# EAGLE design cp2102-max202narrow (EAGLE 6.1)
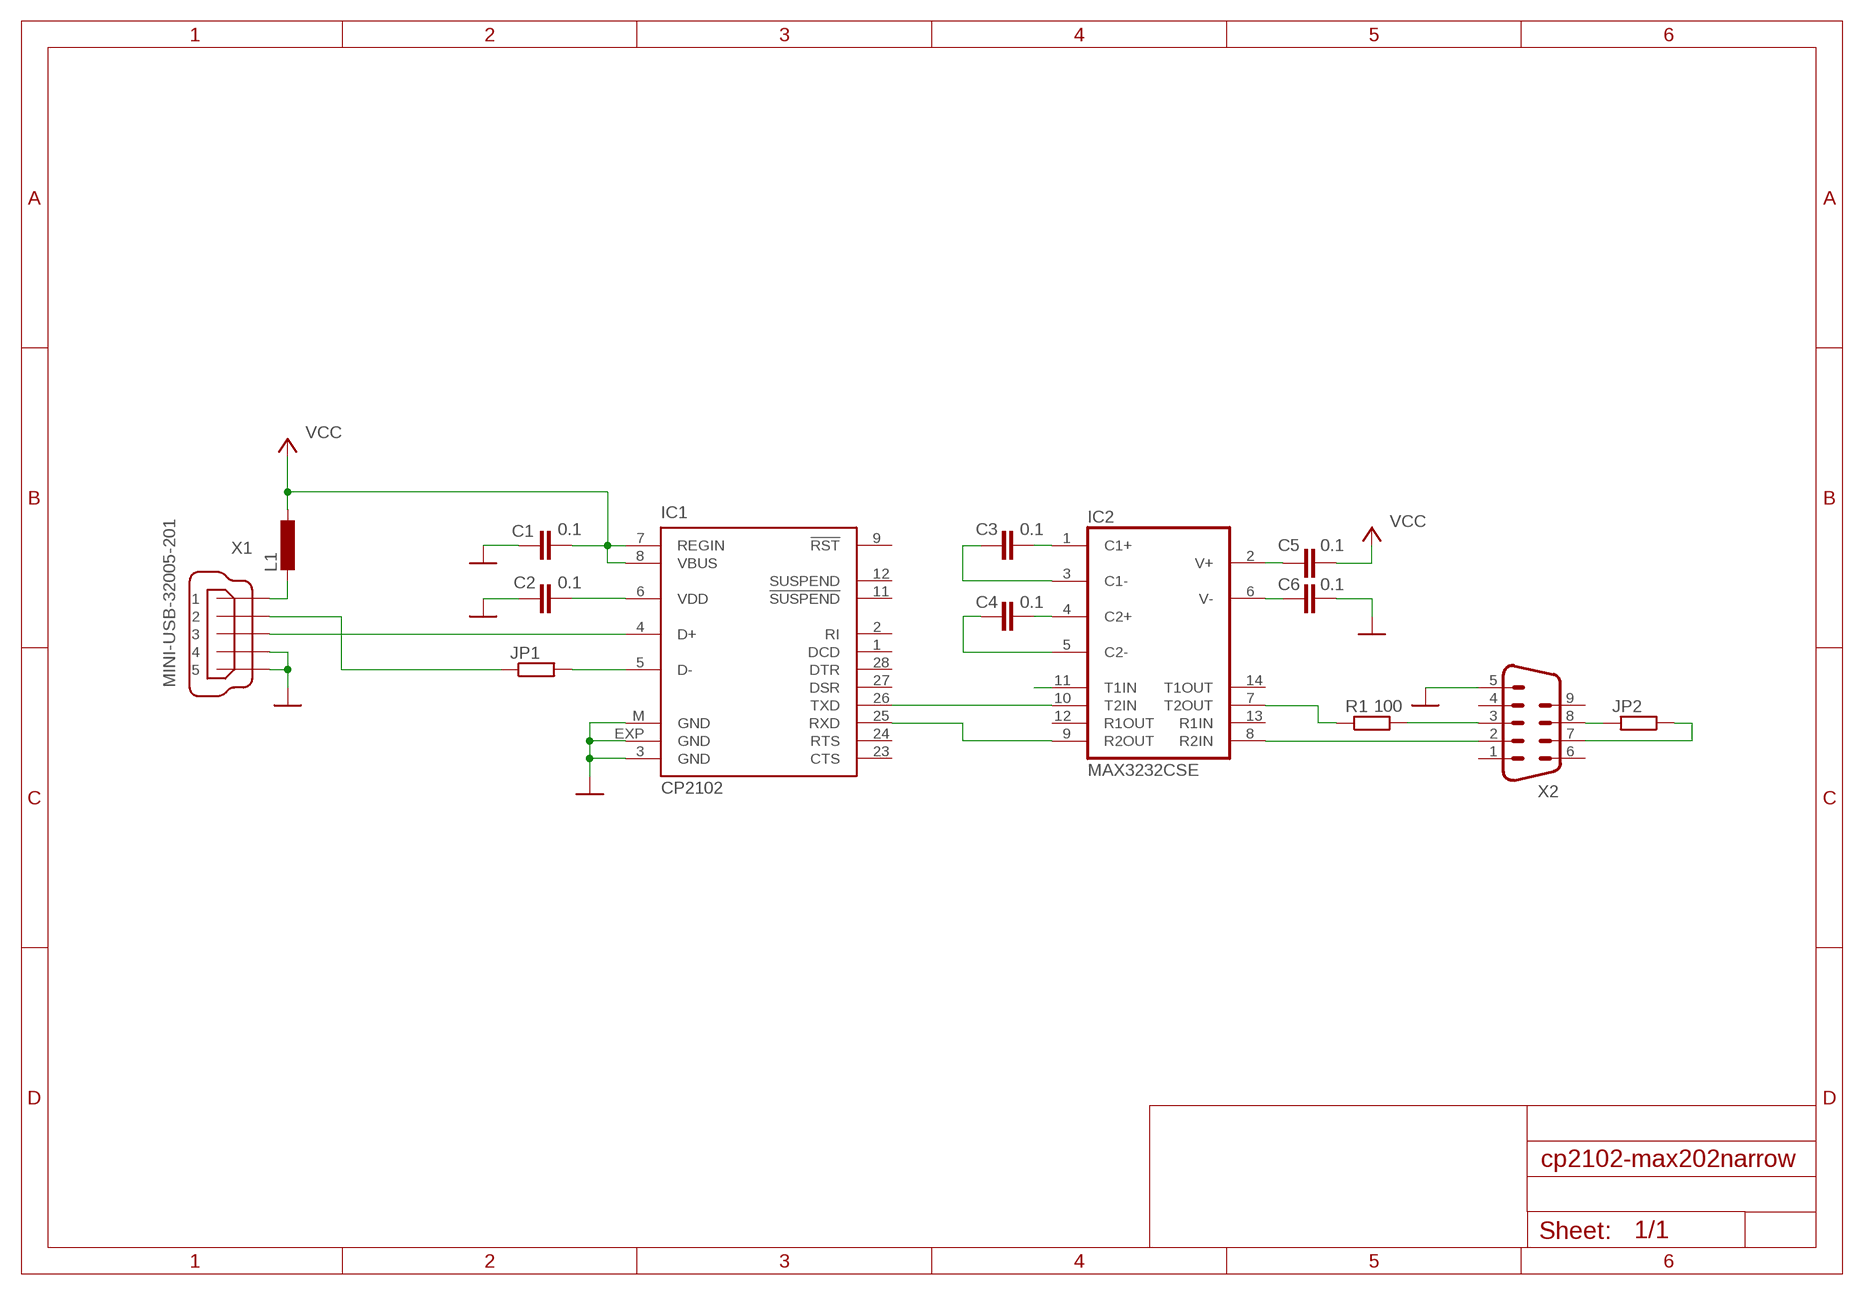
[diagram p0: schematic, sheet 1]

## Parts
C1  0.1  C-EUC0805  [C0805]
C2  0.1  C-EUC0805  [C0805]
C3  0.1  C-EUC0805  [C0805]
C4  0.1  C-EUC0805  [C0805]
C5  0.1  C-EUC0805  [C0805]
C6  0.1  C-EUC0805  [C0805]
IC1  CP2102  [MLP28]
IC2  MAX3232CSE  [SO16]
JP1  R-EU_MELF0102W  [MINI_MELF-0102W]
JP2  R-EU_R0805  [R0805]
L1  L-EUL3216C  [L3216C]
R1  100  R-EU_R0805  [R0805]
X1  MINI-USB-32005-201  [32005-201]
X2  M09D  [M09D]

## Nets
GND: C1.2 C2.2 C6.2 IC1.3(GND) IC1.EXP(GND) IC1.M(GND) X1.4 X1.5 X2.5
N$1: C5.1 IC2.2(V+)
N$2: C6.1 IC2.6(V-)
N$3: C3.2 IC2.1(C1+)
N$4: C3.1 IC2.3(C1-)
N$5: C4.1 IC2.5(C2-)
N$6: C4.2 IC2.4(C2+)
N$7: IC2.8(R2IN) X2.2
N$8: IC2.7(T2OUT) R1.1
N$9: IC1.26(TXD) IC2.10(T2IN)
N$10: IC1.25(RXD) IC2.9(R2OUT)
N$11: C2.1 IC1.6(VDD)
N$12: IC1.5(D-) JP1.2
N$13: IC1.4(D+) X1.3
N$14: L1.2 X1.1
N$15: JP1.1 X1.2
N$16: JP2.2 X2.8
N$17: JP2.1 X2.7
N$18: IC2.11(T1IN)
N$19: R1.2 X2.3
VCC: C1.1 C5.2 IC1.7(REGIN) IC1.8(VBUS) L1.1
Unconnected: IC1.1(DCD) IC1.2(RI) IC1.9(!RST) IC1.11(!SUSPEND) IC1.12(SUSPEND) IC1.23(CTS) IC1.24(RTS) IC1.27(DSR) IC1.28(DTR) IC2.12(R1OUT) IC2.13(R1IN) IC2.14(T1OUT) X2.1 X2.4 X2.6 X2.9

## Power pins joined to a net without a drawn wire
GND: IC2.15(GND)
VCC: IC2.16(VCC)

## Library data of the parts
C1-C6 = rcl:C-EU: CAPACITOR, European symbol
IC1 = silabs:CP210*: Single-Chip USB to UART Bridge Source: www.silabs.com .. CP2101.pdf / cp2102.pdf; MF: FARNELL; MPN: CP2102-GM; OC_FARNELL: 9282130; OC_NEWARK: 30K5635
IC2 = maxim:MAX3232*: True RS-232 Transceivers 3.0V to 5.5V, Low-Power up to 1Mbps, Using Four 0.1µF External Capacitors Source: http://pdfserv.maxim-ic.com/en/ds/MAX3222-MAX3241.pdf; MPN: MAX3232CSE; OC_FARNELL: 9725490; OC_NEWARK: 90C2890
JP1 JP2 R1 = rcl:R-EU_: RESISTOR, European symbol
L1 = rcl:L-EU: INDUCTOR, European symbol
X1 = con-cypressindustries:MINI-USB-: MINI USB-B Conector Source: www.cypressindustries.com; OC_FARNELL: unknown; OC_NEWARK: unknown
X2 = con-subd:M09: SUB-D; OC_FARNELL: unknown; OC_NEWARK: unknown

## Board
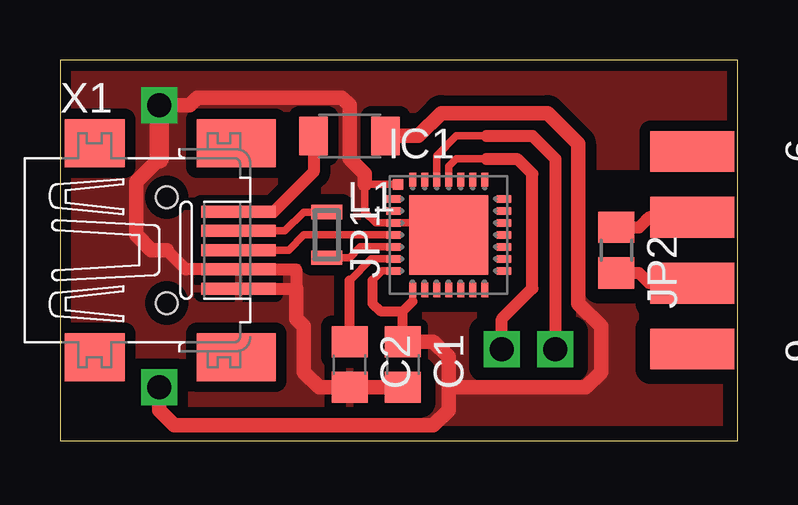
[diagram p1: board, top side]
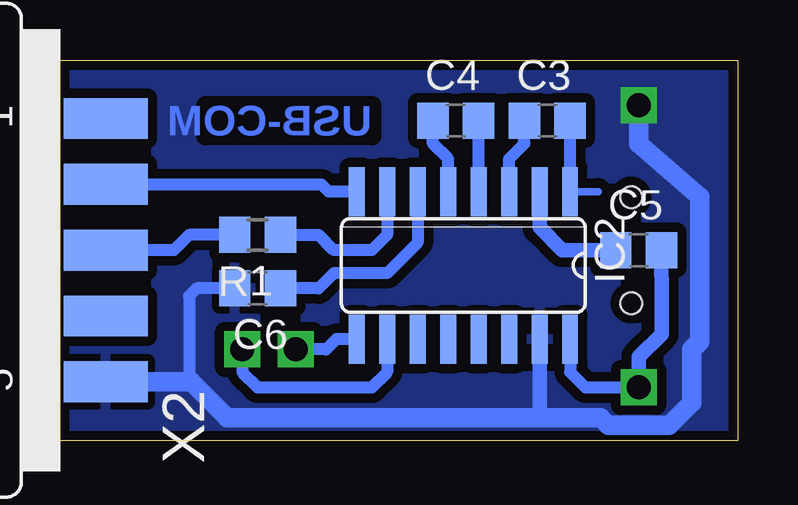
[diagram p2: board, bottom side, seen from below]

Size 28.24 x 15.86 mm. Coordinates in mm from the lower left corner, seen from the top.
Outline: 0,0 28.24,0 28.24,15.86 0,15.86 0,0
Copper layers (1*16): Top 0.035mm / dielectric 1.5mm / Bottom 0.035mm
Design rules: minimum track width 10mil, minimum drill 24mil, track to track 6mil, track to pad 6mil, pad to pad 6mil, via to via 6mil, smd to smd 6mil, copper to edge 5mil, drill to drill 8mil, minimum pad ring 15mil, minimum via ring 8mil, stop-mask expansion 4mil, vias tented up to drill 0mil, thermal gap 12mil

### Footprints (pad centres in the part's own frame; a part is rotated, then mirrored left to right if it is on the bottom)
C0805 = smd 1.3 x 1.5: 1 -0.95,0; 2 0.95,0
MLP28 = smd 0.6 x 0.3: 1 -2.3,1.5; 2 -2.3,1; 3 -2.3,0.5; 4 -2.3,0; 5 -2.3,-0.5; 6 -2.3,-1; 7 -2.3,-1.5; 15 2.3,-1.5; 16 2.3,-1; 17 2.3,-0.5; 18 2.3,0; 19 2.3,0.5; 20 2.3,1; 21 2.3,1.5 | smd 0.3 x 0.6: 8 -1.5,-2.3; 9 -1,-2.3; 10 -0.5,-2.3; 11 0,-2.3; 12 0.5,-2.3; 13 1,-2.3; 14 1.5,-2.3; 22 1.5,2.3; 23 1,2.3; 24 0.5,2.3; 25 0,2.3; 26 -0.5,2.3; 27 -1,2.3; 28 -1.5,2.3 | smd 3.3 x 3.3: EXP 0,0 | smd 0.435 x 0.435: M -2.103,2.103
SO16 = smd 0.66 x 2.032: 1 -4.445,-3.073; 2 -3.175,-3.073; 3 -1.905,-3.073; 4 -0.635,-3.073; 5 0.635,-3.073; 6 1.905,-3.073; 7 3.175,-3.073; 8 4.445,-3.073; 9 4.445,3.073; 10 3.175,3.073; 11 1.905,3.073; 12 0.635,3.073; 13 -0.635,3.073; 14 -1.905,3.073; 15 -3.175,3.073; 16 -4.445,3.073
MINI_MELF-0102W = smd 0.6 x 1.3: 1 -0.95,0; 2 0.95,0
R0805 = smd 1.3 x 1.5: 1 -0.95,0; 2 0.95,0
L3216C = smd 1.2 x 1.6: 1 -1.5,0; 2 1.5,0
32005-201 = smd 3.1 x 0.5: 1 3,1.6; 2 3,0.8; 3 3,0; 4 3,-0.8; 5 3,-1.6 | smd 2.5 x 2: M1 -3,-4.45; M2 -3,4.45 | smd 3.3 x 2: M3 2.9,4.45; M4 2.9,-4.45 | hole 0.9: 0,2.2; 0,-2.2
M09D = smd 1.7 x 3.5: 1 5.486,-6.045; 2 2.743,-6.045; 3 0,-6.045; 4 -2.743,-6.045; 5 -5.486,-6.045 | smd 1.7 x 3.5 bottom: 6 4.115,-6.045; 7 1.372,-6.045; 8 -1.372,-6.045; 9 -4.115,-6.045

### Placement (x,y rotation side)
C1  14.29,3.17 270 top
C2  12.06,3.17 270 top
C3  7.94,13.34 0 bottom
C4  11.75,13.34 0 bottom
C5  4.13,7.94 0 bottom
C6  20,6.35 180 bottom
IC1  16.19,8.57 0 top
IC2  11.43,7.3 180 bottom
JP1  11.11,8.57 270 top
JP2  23.18,7.94 270 top
L1  12.06,12.7 180 top
R1  20,8.57 180 bottom
X1  4.45,7.94 0 top
X2  32.38,7.94 90 bottom

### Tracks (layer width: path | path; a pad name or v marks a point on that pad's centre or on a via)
GND  (via drill 1)
  Top 0.32: IC1.EXP 16.19,9.07 IC1.3 13.15,9.07 12.7,9.53 12.7,10.68 IC1.M
  Top 0.5: X1.5 9.84,6.34 9.84,7.14 X1.4 5.25,7.14 4.45,7.94
  Top 0.61: 12.7,10.68 12.7,11.11 12.06,11.75 12.06,13.97 11.75,14.29 5.71,14.29 5.4,13.97 v4.13,13.97 | 4.13,11.75 3.17,10.79 3.17,8.57 3.81,7.94 4.45,7.94 | C1.2 C2.2 10.79,2.22 10.16,2.86 10.16,4.76 9.84,5.08 9.84,6.34
  Top 0.813: 4.13,11.75 v4.13,13.97
  Bottom 0.5: C6.2 22.54,6.35 22.86,6.03 22.86,2.45
  Bottom 0.61: IC2.15 8.26,0.95
  Bottom 0.813: v4.13,13.97 4.13,12.38 1.59,10.16 1.59,4.13 1.91,3.81 1.91,1.59 2.86,0.64 5.4,0.64 5.71,0.95 8.26,0.95 21.27,0.95 22.77,2.45 22.86,2.45 X2.5
  pour Top (isolate 0.45): -6.99,18.73 -6.99,-3.17 12.38,-3.17 12.38,12.06 20.95,12.06 20.95,11.43 38.73,11.43 38.73,18.73
  pour Bottom (isolate 0.4): -7.62,17.78 43.18,17.78 43.18,-2.54 -7.62,-2.54
N$1
  Bottom 0.61: C5.1 7.3,7.94 8.26,8.89 IC2.2
N$2
  Bottom 0.5: IC2.6 13.34,8.26 14.61,6.99 16.83,6.99 17.46,6.35 C6.1
N$3
  Bottom 0.32: IC2.1 5.82,10.38
  Bottom 0.5: IC2.1 6.99,13.02 C3.2
N$4
  Bottom 0.5: IC2.3 9.53,11.75 8.89,12.38 C3.1
N$5
  Bottom 0.5: IC2.5 12.06,11.75 12.7,12.38 12.7,13.02 C4.1
N$6
  Bottom 0.5: IC2.4 C4.2
N$7
  Bottom 0.5: IC2.8 17.04,10.38 17.35,10.68 X2.2
N$8
  Bottom 0.5: IC2.7 14.61,8.57 15.24,7.94 16.83,7.94 17.46,8.57 R1.1
N$9  (via drill 1)
  Top 0.32: IC1.26 15.69,11.88 16.51,12.7 17.78,12.7
  Top 0.5: 17.78,12.7 19.68,12.7 20.64,11.75 v20.64,3.81
  Bottom 0.5: v20.64,3.81 20.64,2.86 20,2.22 15.24,2.22 14.61,2.86 IC2.10
N$10  (via drill 1)
  Top 0.32: IC1.25 16.19,11.43 16.51,11.75 17.78,11.75
  Top 0.5: v18.41,3.81 18.41,5.08 19.68,6.35 19.68,11.11 19.05,11.75 17.78,11.75
  Bottom 0.5: 15.88,3.81 IC2.9 16.73,4.23 17.14,3.81 v18.41,3.81
N$11
  Top 0.32: IC1.6 12.97,7.57 12.06,6.67
  Top 0.406: C2.1 12.06,6.67
N$12
  Top 0.32: IC1.5 12.52,8.07 12.07,7.62 JP1.2
N$13
  Top 0.32: IC1.4 10.16,8.57 9.53,7.94 X1.3
N$14
  Top 0.5: X1.1 8.9,9.54 10.56,11.2 L1.2
N$15
  Top 0.32: X1.2 9.37,8.74 10.16,9.52 JP1.1
N$16
  Top 0.5: X2.8 24.55,6.57 24.13,6.99 JP2.2
  Top 0.61: JP2.2
N$17
  Top 0.5: X2.7 24.55,9.31 24.45,9.21 24.13,8.89 JP2.1
N$19
  Bottom 0.5: R1.2 22.86,8.57 23.5,7.94 X2.3
VCC  (via drill 1)
  Top 0.32: IC1.7 13.42,7.07 13.02,6.67 | IC1.8 14.69,5.8
  Top 0.406: 13.02,6.67 13.02,5.71 13.34,5.4 14.29,5.4 | 14.29,5.4 14.69,5.8 | C1.1 14.29,5.4
  Top 0.61: v4.13,2.22 4.13,1.27 4.76,0.64 15.56,0.64 16.19,1.27 16.19,2.22 | L1.1 14.92,12.7 15.88,13.65 20.32,13.65 21.59,12.38 21.59,5.71 22.54,4.76 22.54,2.86 21.91,2.22 16.19,2.22 | 16.19,2.22 16.19,3.49 15.56,4.12 C1.1
  Bottom 0.5: IC2.16 6.99,2.86 6.35,2.22 v4.13,2.22
  Bottom 0.61: v4.13,2.22 4.13,3.49 3.17,4.45 3.17,6.67 3.18,6.99 C5.2
  pour Top (isolate 0.61): 15.24,-1.27 15.24,6.99 30.48,6.99 30.48,-1.27

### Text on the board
Bottom: USB-COM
